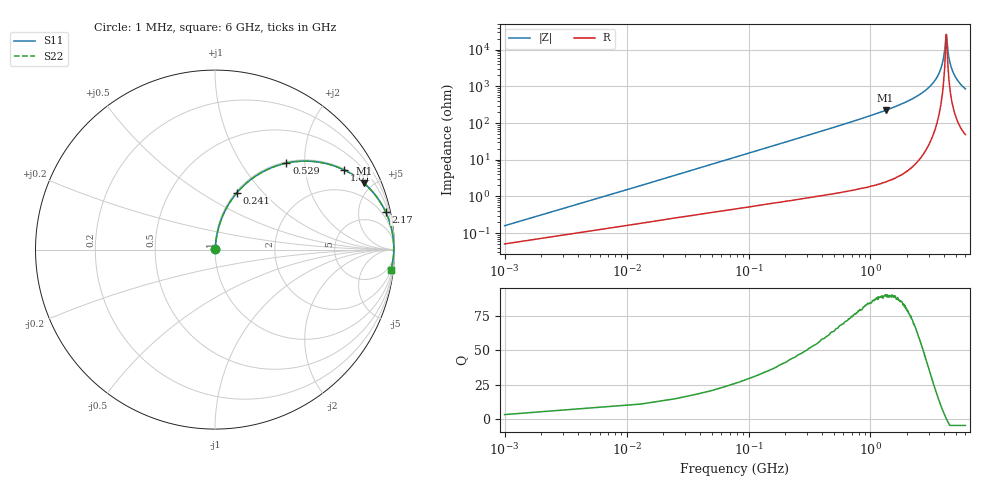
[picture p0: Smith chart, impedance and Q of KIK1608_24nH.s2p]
!version-2
!date-01.2022
!Series
# MHz S RI R 50
!Freq ReS11 ImS11 ReS21 ImS21 ReS12 ImS12 ReS22 ImS22
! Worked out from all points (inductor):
!   501 points, 1 MHz to 6 GHz, reference 50 ohm
!   read as one part in series: L = 24 nH near 25 MHz
!   highest Q = 89.9 at 1.33 GHz (marker M1), where L = 26.8 nH
!   self-resonance near 4.18 GHz
!   S11 on the Smith chart (normalised r, x): 1 MHz: 1.00, +0.00; 241 MHz: 1.02, +0.73; 529 MHz: 1.02, +1.62; 1.01 GHz: 1.04, +3.23; 2.17 GHz: 1.12, +8.97; 6 GHz: 2, -17
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1  0.000518 0.00151  0.9995 -0.00151  0.9995 -0.00151  0.000518 0.00151
37  0.00621 0.0553  0.9938 -0.0553  0.9938 -0.0553  0.00621 0.0553
61  0.0123 0.0905  0.9877 -0.0905  0.9877 -0.0905  0.0123 0.0905
133  0.044 0.1908  0.956 -0.1908  0.956 -0.1908  0.044 0.1908
241  0.1228 0.3173  0.8772 -0.3173  0.8772 -0.3173  0.1228 0.3173
529  0.3981 0.482  0.6019 -0.482  0.6019 -0.482  0.3981 0.482
1010  0.7207 0.4428  0.2793 -0.4428  0.2793 -0.4428  0.7207 0.4428
1330  0.8307 0.3695  0.1693 -0.3695  0.1693 -0.3695  0.8307 0.3695
2020  0.9375 0.2359  0.0625 -0.2359  0.0625 -0.2359  0.9375 0.2359
2170  0.9501 0.2111  0.05 -0.2111  0.05 -0.2111  0.9501 0.2111
3010  0.9861 0.1042  0.0139 -0.1042  0.0139 -0.1042  0.9861 0.1042
3640  0.9948 0.0443  0.00524 -0.0443  0.00524 -0.0443  0.9948 0.0443
3880  0.9959 0.0241  0.00407 -0.0241  0.00407 -0.0241  0.9959 0.0241
4010  0.9962 0.0136  0.0038 -0.0136  0.0038 -0.0136  0.9962 0.0136
4110  0.9963 0.00612  0.00375 -0.00612  0.00375 -0.00612  0.9963 0.00612
4160  0.9962 0.00156  0.00378 -0.00156  0.00378 -0.00156  0.9962 0.00156
4190  0.9962 -0.000246  0.0038 0.000246  0.0038 0.000246  0.9962 -0.000246
4330  0.9959 -0.0109  0.00409 0.0109  0.00409 0.0109  0.9959 -0.0109
4450  0.9955 -0.0194  0.00449 0.0194  0.00449 0.0194  0.9955 -0.0194
4700  0.9942 -0.0367  0.0058 0.0367  0.0058 0.0367  0.9942 -0.0367
5010  0.9919 -0.0562  0.00805 0.0562  0.00805 0.0562  0.9919 -0.0562
6000  0.9803 -0.1134  0.0197 0.1134  0.0197 0.1134  0.9803 -0.1134
